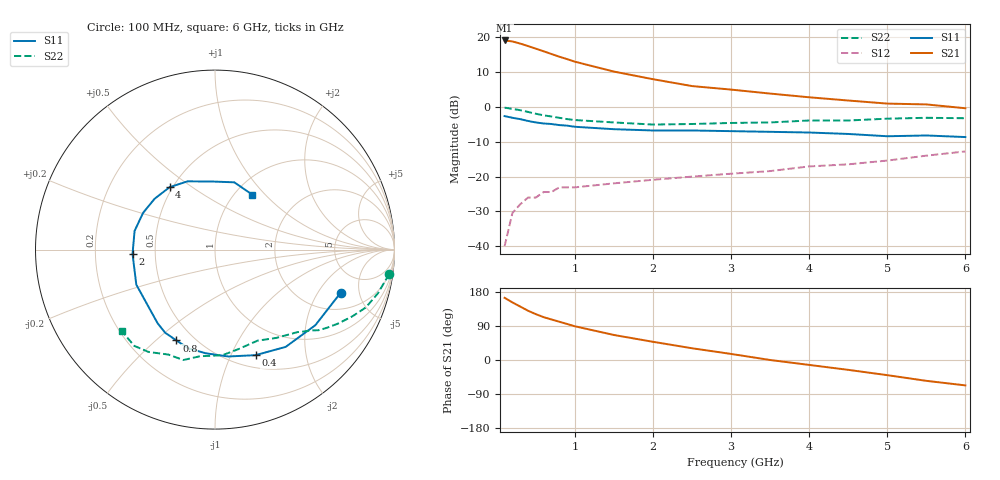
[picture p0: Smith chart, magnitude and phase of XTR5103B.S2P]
! HXTR-5103  (2N6741) Common Emitter
! Vce=15V  Ic=15mA
# ghz s ma r 50
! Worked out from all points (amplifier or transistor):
!   20 points, 100 MHz to 6 GHz, reference 50 ohm
!   highest |S21| = 19.1 dB at 100 MHz (marker M1)
!   |S21| within 3 dB of that: start of sweep to 584.4 MHz
!   unconditionally stable (mu >= 1): 1.673 GHz to 5.106 GHz
!   at 400 MHz: K = 0.34, MSG = 21.8 dB, |S12| = -26.0 dB
!   at 1.5 GHz: K = 0.93, MSG = 16.1 dB, |S12| = -21.9 dB
!   at 6 GHz: K = 0.88, MSG = 6.2 dB, |S12| = -12.8 dB
!   S11 on the Smith chart (normalised r, x): 100 MHz: 3.05, -3.25; 400 MHz: 0.64, -1.24; 800 MHz: 0.40, -0.58; 2 GHz: 0.37, -0.02; 4 GHz: 0.48, +0.41; 6 GHz: 1.19, +0.85
0.1  0.74 -19.0  9.05 164.0  0.01 81.0  0.98 -8.0
0.2  0.7 -37.0  8.76 152.0  0.03 68.0  0.94 -15.0
0.3  0.67 -54.0  8.16 141.0  0.04 60.0  0.9 -21.0
0.4  0.63 -69.0  7.52 130.0  0.05 53.0  0.85 -26.0
0.5  0.6 -83.0  6.9 121.0  0.05 48.0  0.8 -31.0
0.6  0.58 -95.0  6.32 113.0  0.06 43.0  0.76 -35.0
0.7  0.57 -105.0  5.78 107.0  0.06 40.0  0.73 -38.0
0.8  0.55 -113.0  5.29 101.0  0.07 37.0  0.7 -40.0
0.9  0.54 -121.0  4.88 95.0  0.07 34.0  0.67 -43.0
1  0.52 -128.0  4.48 89.0  0.07 31.0  0.65 -45.0
1.5  0.48 -156.0  3.23 66.0  0.08 25.0  0.6 -55.0
2  0.46 -177.0  2.51 48.0  0.09 21.0  0.56 -65.0
2.5  0.46 167.0  2 31.0  0.1 18.0  0.57 -77.0
3  0.45 153.0  1.78 16.0  0.11 16.0  0.59 -86.0
3.5  0.44 140.0  1.56 0.0  0.12 12.0  0.6 -98.0
4  0.43 126.0  1.38 -13.0  0.14 8.0  0.64 -106.0
4.5  0.41 112.0  1.24 -26.0  0.15 4.0  0.64 -114.0
5  0.38 93.0  1.12 -40.0  0.17 -1.0  0.68 -123.0
5.5  0.39 74.0  1.09 -55.0  0.2 -6.0  0.7 -130.0
6  0.37 56.0  0.96 -67.0  0.23 -12.0  0.69 -139.0
